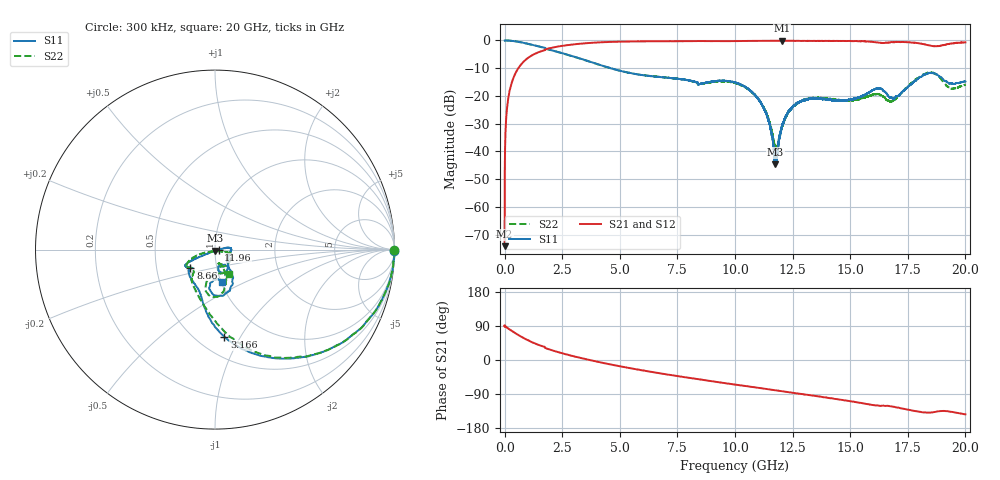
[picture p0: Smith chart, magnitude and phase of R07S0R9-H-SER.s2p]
!{R07S0R9}
!Johanson Technology Inc.
!www.johansontechnology.com
!Test Board Conditions:
!Substrate Type  RO4350B
!Substrate Thickness  10 mil
!Substrate Dk  3.66
!TL Type: GCPW
!TL Trace Width  21 mil
!TL Gap  20 mil
!Electrode orientation  Horizontal
!DUT TOPOLOGY	SERIES
!Mounting Pad LxW  16x21 mil
! Created Fri Feb  5 23:07:41 2021
# hz S ma R 50
! 2 Port Network Data from SP1.SP block
! freq  magS11  angS11  magS21  angS21  magS12  angS12  magS22  angS22
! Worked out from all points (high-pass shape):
!   20001 points, 300 kHz to 20 GHz, reference 50 ohm
!   highest |S21| = -0.08 dB at 12.04 GHz (marker M1); lowest = -74.1 dB at 300 kHz (marker M2)
!   |S21| within 3 dB of the highest: 1.833 GHz to end of sweep
!   lowest |S11| = -44.6 dB at 11.76 GHz (marker M3), VSWR 1.01, Z = 50.1 - j0.584 ohm
!   |S11| at or under -10 dB: 4.603454 GHz to 4.606218 GHz (2.763 MHz wide, 0.06 % of centre); 4.606 GHz to end of sweep
!   |S22| runs from -41.4 to 0.0 dB; largest |S21 - S12| = 0.011
!   S11 on the Smith chart (normalised r, x): 300 kHz: open; 3.166 GHz: 0.67, -0.86; 8.66 GHz: 0.74, -0.15; 11.96 GHz: 1.04, +0.00; 20 GHz: 1.02, -0.38
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300000  0.9974 -0.4  0.0001965 90.5  0.0002085 70.2  1 -0.3
1.013e8  0.9954 -4.1  0.05805 85.6  0.0581 85.6  0.9965 -4.3
1.313e8  0.9969 -5.5  0.07531 84.3  0.07515 84.4  0.997 -5.5
4.853e8  0.9617 -19.4  0.2629 70.1  0.2625 70.0  0.9612 -19.6
1.4883e9  0.7797 -50.0  0.6172 39.6  0.617 39.5  0.7791 -50.0
3.1663e9  0.4883 -83.8  0.8665 7.5  0.8654 7.4  0.4871 -80.7
3.3343e9  0.4648 -86.4  0.8789 4.9  0.878 5.0  0.462 -83.2
6.6673e9  0.2206 -121.8  0.9669 -34.3  0.9677 -34.3  0.2217 -125.0
8.6603e9  0.1705 -143.8  0.9754 -52.8  0.9734 -52.9  0.1685 -142.4
1.00003e10  0.176 -153.5  0.9747 -64.8  0.9747 -64.8  0.171 -154.3
1.11613e10  0.06999 -153.6  0.986 -74.7  0.986 -74.7  0.07167 -163.3
1.14723e10  0.03418 -149.3  0.988 -77.5  0.9876 -77.5  0.03621 -159.5
1.17573e10  0.005893 -81.6  0.9885 -80.0  0.9886 -79.9  0.01156 -104.9
1.19583e10  0.02006 1.5  0.9872 -81.7  0.9867 -81.7  0.02011 -29.6
1.20353e10  0.02866 4.3  0.9904 -82.4  0.9896 -82.4  0.02736 -19.7
1.25453e10  0.06689 7.5  0.9871 -86.9  0.9863 -86.7  0.06712 -13.4
1.33343e10  0.09042 2.1  0.9819 -93.6  0.9804 -93.6  0.09175 -15.3
1.62263e10  0.1357 -67.1  0.9119 -120.3  0.9109 -120.4  0.1083 -58.8
1.66673e10  0.09783 -79.2  0.9104 -121.1  0.9132 -121.4  0.08262 -77.8
1.83793e10  0.2554 -77.7  0.8236 -138.9  0.8261 -138.9  0.2627 -87.0
1.93673e10  0.1696 -90.5  0.881 -136.7  0.8838 -136.5  0.1361 -84.5
2e10  0.1832 -77.1  0.9232 -143.5  0.922 -143.5  0.1601 -59.6
